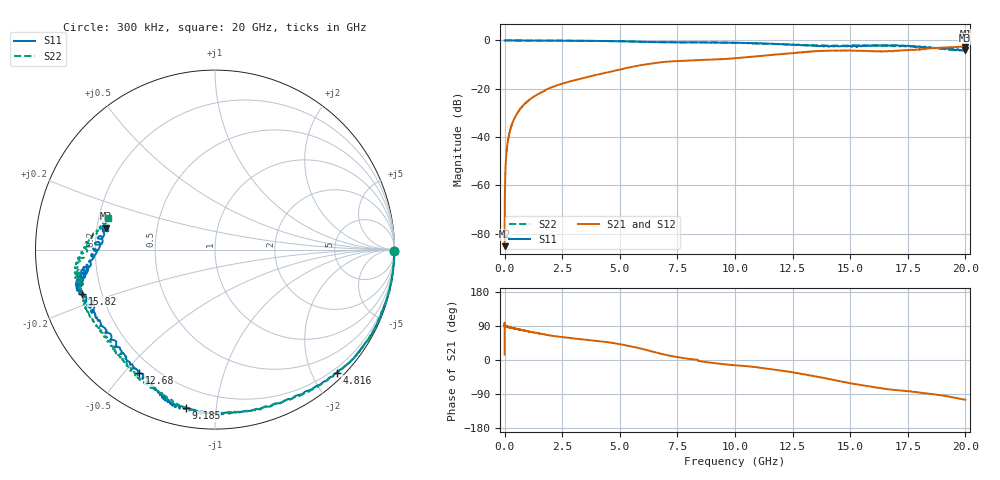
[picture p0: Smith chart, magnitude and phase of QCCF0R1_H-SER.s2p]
!{QCCF0R1}
!Johanson Technology Inc.
!www.johansontechnology.com
!Test Board Conditions:
!Substrate Type  RO4350B
!Substrate Thickness  10 mil
!Substrate Dk  3.66
!TL Type: GCPW
!TL Trace Width  21 mil
!TL Gap  20 mil
!Electrode orientation  Horizontal
!DUT TOPOLOGY	SERIES
!Mounting Pad LxW  16x21 mil
! Created Sat Jan  9 18:09:07 2021
# hz S ma R 50
! 2 Port Network Data from SP1.SP block
! freq  magS11  angS11  magS21  angS21  magS12  angS12  magS22  angS22
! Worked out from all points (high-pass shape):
!   20001 points, 300 kHz to 20 GHz, reference 50 ohm
!   highest |S21| = -2.52 dB at 20 GHz (marker M1); lowest = -85.2 dB at 300 kHz (marker M2)
!   |S21| within 3 dB of the highest: 12.15 GHz to 12.21 GHz (68.13 MHz wide, 0.559 % of centre); 12.21 GHz to end of sweep
!   lowest |S11| = -4.1 dB at 20 GHz (marker M3), VSWR 4.28, Z = 11.8 + j4.6 ohm
!   |S11| at or under -10 dB: nowhere
!   |S22| runs from -4.2 to 0.0 dB; largest |S21 - S12| = 0.024
!   S11 on the Smith chart (normalised r, x): 300 kHz: open; 4.816 GHz: 0.12, -2.39; 9.185 GHz: 0.09, -0.83; 12.68 GHz: 0.14, -0.55; 15.82 GHz: 0.13, -0.16; 20 GHz: 0.24, +0.09
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300000  0.9987 -0.4  5.472e-05 14.2  4.371e-05 53.8  0.9992 -0.5
1.063e8  0.9991 -1.5  0.006086 87.9  0.006148 88.7  0.9999 -1.5
1.563e8  0.9976 -2.4  0.008924 87.2  0.008957 87.1  0.9976 -2.3
3.113e8  0.999 -4.4  0.01773 84.9  0.01772 84.7  0.9989 -4.6
5.643e8  0.9994 -8.0  0.03197 81.5  0.03186 81.6  0.9989 -8.1
1.0573e9  0.9968 -14.4  0.05816 75.4  0.05803 75.2  0.9962 -14.5
1.8503e9  0.9923 -23.8  0.09805 65.7  0.09801 65.9  0.9916 -23.9
3.3343e9  0.9853 -35.3  0.1626 54.6  0.1635 54.7  0.985 -34.6
4.8163e9  0.9648 -45.4  0.2385 43.6  0.2383 43.9  0.962 -46.0
5.7303e9  0.9446 -55.7  0.2971 32.8  0.2973 32.8  0.9443 -57.5
6.6673e9  0.9261 -70.8  0.3476 18.2  0.3495 18.6  0.9188 -71.5
8.2863e9  0.9201 -91.1  0.3888 1.0  0.3907 1.4  0.9086 -86.0
8.4873e9  0.912 -92.4  0.3927 -3.1  0.3941 -3.0  0.9115 -93.3
9.1853e9  0.8983 -100.5  0.4054 -8.9  0.4053 -9.4  0.9132 -97.2
1.00003e10  0.895 -105.2  0.4294 -13.9  0.428 -13.6  0.8941 -101.5
1.26783e10  0.8058 -121.5  0.5573 -34.4  0.56 -35.2  0.8119 -126.8
1.33343e10  0.7864 -129.3  0.5923 -41.4  0.5917 -41.8  0.7912 -132.9
1.58193e10  0.778 -161.7  0.6028 -69.6  0.601 -69.7  0.7828 -158.2
1.66673e10  0.7928 -163.7  0.6028 -77.3  0.5968 -75.6  0.7861 -169.2
1.85513e10  0.7004 -172.6  0.6915 -89.9  0.6872 -89.0  0.7047 174.9
1.99963e10  0.6212 168.9  0.746 -104.9  0.7499 -104.5  0.6194 163.2
2e10  0.6216 168.8  0.748 -105.0  0.7512 -104.4  0.6199 163.2
